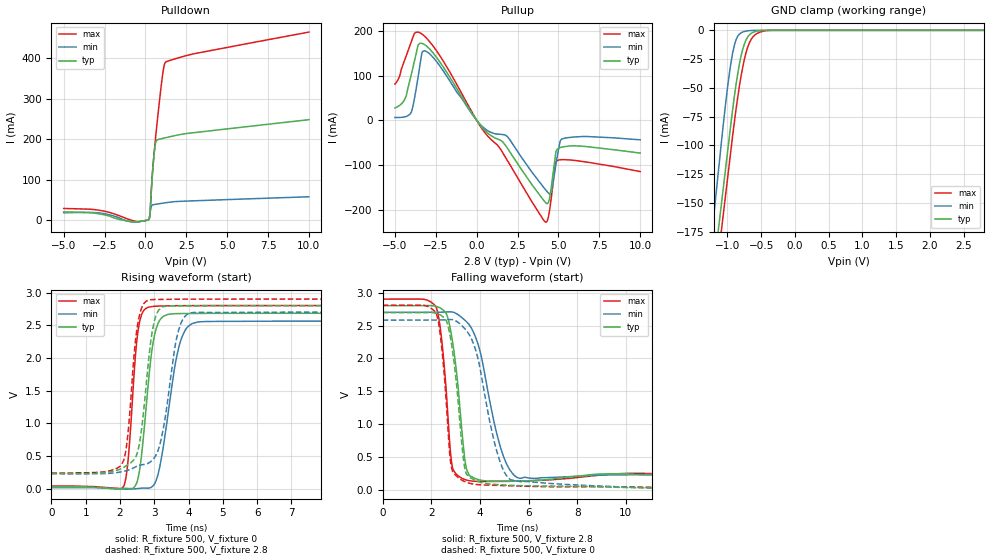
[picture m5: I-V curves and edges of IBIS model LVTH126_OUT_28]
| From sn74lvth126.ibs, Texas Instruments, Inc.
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[Model]   LVTH126_OUT_28
Model_type  3-state
Enable   Active-High
Vref =   0
Rref =   500
Cref =   50p
Vmeas =   1.5
| variable   typ   min   max
C_comp   3.48pF   2.89pF   4.65pF
| C_pullup   3.98pF   0.17pF   5.57pF
| C_pulldown   4.80pF   0.18pF   12.93pF
| C_tri-state   3.48pF   2.89pF   4.65pF
[Temperature Range]   40   -40   100
| Ambient temperature   25   -40   85
[Voltage range]   2.8   2.7   2.9
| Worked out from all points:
|   slope of the pulldown table from 0 to 0.42 V, typ, clamps not added: 3.84 ohm
|   slope of the pullup table from 0 to 0.42 V, typ, clamps not added: 21.6 ohm
|   GND clamp passes 1 mA (typ) near -0.58 V on its own axis
|   rising waveform, R_fixture 500, V_fixture 0: 20-80 % time 302ps typ, 441ps min, 227ps max; typ from 0.032 V to 2.68 V
|   falling waveform, R_fixture 500, V_fixture 2.8: 20-80 % time 439ps typ, 862ps min, 345ps max; typ from 2.8 V to 0.238 V
|   rising waveform, R_fixture 500, V_fixture 2.8: 20-80 % time 322ps typ, 431ps min, 257ps max; typ from 0.238 V to 2.8 V
|   falling waveform, R_fixture 500, V_fixture 0: 20-80 % time 440ps typ, 874ps min, 345ps max; typ from 2.69 V to 0.032 V
[GND Clamp]
| LVTH126_OUT_28
|   Voltage   I(typ)   I(min)   I(max)
-5.5V     -2.834A    -3.019A    -2.854A
-1.22V    -215.7mA   -171mA     -239.3mA
-1.18V    -195.7mA   -148.2mA   -219mA
-1.075V   -143.6mA   -88.89mA   -166.6mA
-975mV    -94.01mA   -38.86mA   -117.1mA
-925mV    -69.63mA   -20.27mA   -92.47mA
-875mV    -47.88mA   -8.568mA   -69.46mA
-800mV    -22.55mA   -2.203mA   -40.18mA
-725mV    -8.33mA    -701.6uA   -19.48mA
-650mV    -2.727mA   -178.1uA   -7.97mA
-575mV    -842.6uA   -11.41uA   -3.176mA
2.8V      28.19pA    20.95pA    1.193nA
[Pulldown]
| LVTH126_OUT_28
|   Voltage   I(typ)   I(min)   I(max)
-5V       21.12mA    18.87mA    29.39mA
-2.715V   15.38mA    17.88mA    24.31mA
-705mV    -3.568mA   -4.339mA   -1.2mA
215mV     2.333mA    2.789mA    2.244mA
285mV     22.67mA    17.64mA    18.47mA
365mV     76.41mA    34.67mA    76.09mA
465mV     132.9mA    38.48mA    134.9mA
620mV     189.7mA    39.59mA    203.1mA
1.045V    201.8mA    42.37mA    356.7mA
1.15V     202.8mA    43.01mA    381.7mA
1.255V    203.9mA    43.63mA    390.3mA
10V       248mA      58.23mA    463.7mA
[Pullup]
| LVTH126_OUT_28
|   Voltage   I(typ)   I(min)   I(max)
-5V       27.58mA    6.461mA    80.9mA
-4.385V   48mA       7.971mA    136.7mA
-3.995V   103.2mA    18.88mA    176mA
-3.58V    167.9mA    97.78mA    196.9mA
-3.205V   169.4mA    155.1mA    188.3mA
115mV     -5.868mA   -5.032mA   -6.972mA
1.865V    -61.28mA   -35.76mA   -88.87mA
4.215V    -183.5mA   -154.8mA   -227.1mA
4.55V     -152.6mA   -160.2mA   -176.4mA
4.945V    -63.72mA   -76.79mA   -89.28mA
5.415V    -58.25mA   -39.36mA   -87.74mA
10V       -72.92mA   -43.35mA   -114.2mA
[Ramp]
| LVTH126_OUT_28
| variable   typ   min   max
dV/dt_r   1.61/3.10E-10   1.54/4.53E-10   1.68/2.33E-10
dV/dt_f   1.60/4.57E-10   1.51/8.91E-10   1.66/3.61E-10
R_load = 500
[Rising Waveform]
| LVTH126_OUT_28
R_fixture =   500
C_fixture =   0
L_fixture =   0
V_fixture =   0
V_fixture_min = 0
V_fixture_max = 0
|   Time   V(typ)   V(min)   V(max)
0s        32.04mV    19.78mV    45.03mV
2.115ns   8.934mV    -2.04mV    44.55mV
2.245ns   7.596mV    -3.124mV   483.9mV
2.44ns    44.18mV    2.652mV    1.959V
2.545ns   205.5mV    7.369mV    2.471V
2.965ns   2.232V     48.63mV    2.788V
3.18ns    2.59V      388.4mV    2.794V
3.745ns   2.678V     2.219V     2.799V
4.32ns    2.681V     2.553V     2.8V
50ns      2.684V     2.563V     2.801V
[Falling Waveform]
| LVTH126_OUT_28
R_fixture =   500
C_fixture =   0
L_fixture =   0
V_fixture =   2.8
V_fixture_min = 2.7
V_fixture_max = 2.9
|   Time   V(typ)   V(min)   V(max)
0s        2.8V       2.7V       2.9V
2.19ns    2.791V     2.701V     2.783V
2.395ns   2.759V     2.702V     2.388V
2.625ns   2.673V     2.706V     1.455V
2.885ns   2.225V     2.703V     326.9mV
3.375ns   481.2mV    2.583V     166.7mV
3.635ns   211mV      2.469V     144.4mV
4.89ns    138.8mV    602.7mV    138.3mV
5.63ns    142.4mV    184.8mV    142.3mV
50ns      237.6mV    231.8mV    243.7mV
[Rising Waveform]
| LVTH126_OUT_28
R_fixture =   500
C_fixture =   0
L_fixture =   0
V_fixture =   2.8
V_fixture_min = 2.7
V_fixture_max = 2.9
|   Time   V(typ)   V(min)   V(max)
0s        238mV      232mV      244.1mV
2.055ns   313.4mV    263.2mV    381.9mV
2.215ns   364mV      283.7mV    756.6mV
2.425ns   457.6mV    329.4mV    2.122V
2.54ns    621.4mV    356.5mV    2.582V
2.9ns     2.26V      419mV      2.89V
3.225ns   2.776V     815.5mV    2.895V
3.705ns   2.795V     2.413V     2.898V
4.135ns   2.797V     2.695V     2.899V
50ns      2.8V       2.7V       2.9V
[Falling Waveform]
| LVTH126_OUT_28
R_fixture =   500
C_fixture =   0
L_fixture =   0
V_fixture =   0
V_fixture_min = 0
V_fixture_max = 0
|   Time   V(typ)   V(min)   V(max)
0s        2.695V     2.582V     2.808V
2.19ns    2.686V     2.583V     2.69V
2.39ns    2.656V     2.583V     2.296V
2.615ns   2.572V     2.588V     1.339V
2.87ns    2.127V     2.589V     296.8mV
3.365ns   363.1mV    2.456V     136.4mV
3.745ns   164.3mV    2.216V     95.88mV
4.815ns   87.39mV    451.4mV    75.73mV
5.67ns    73.02mV    132.7mV    65.88mV
50ns      32.07mV    19.8mV     45.08mV
